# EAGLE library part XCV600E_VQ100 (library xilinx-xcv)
xcv600e_vq100 edit this description Auto generated by make-symbol-device-package-bsdl.ulp Rev. 26 Source: xcv600e_vq100.bsd
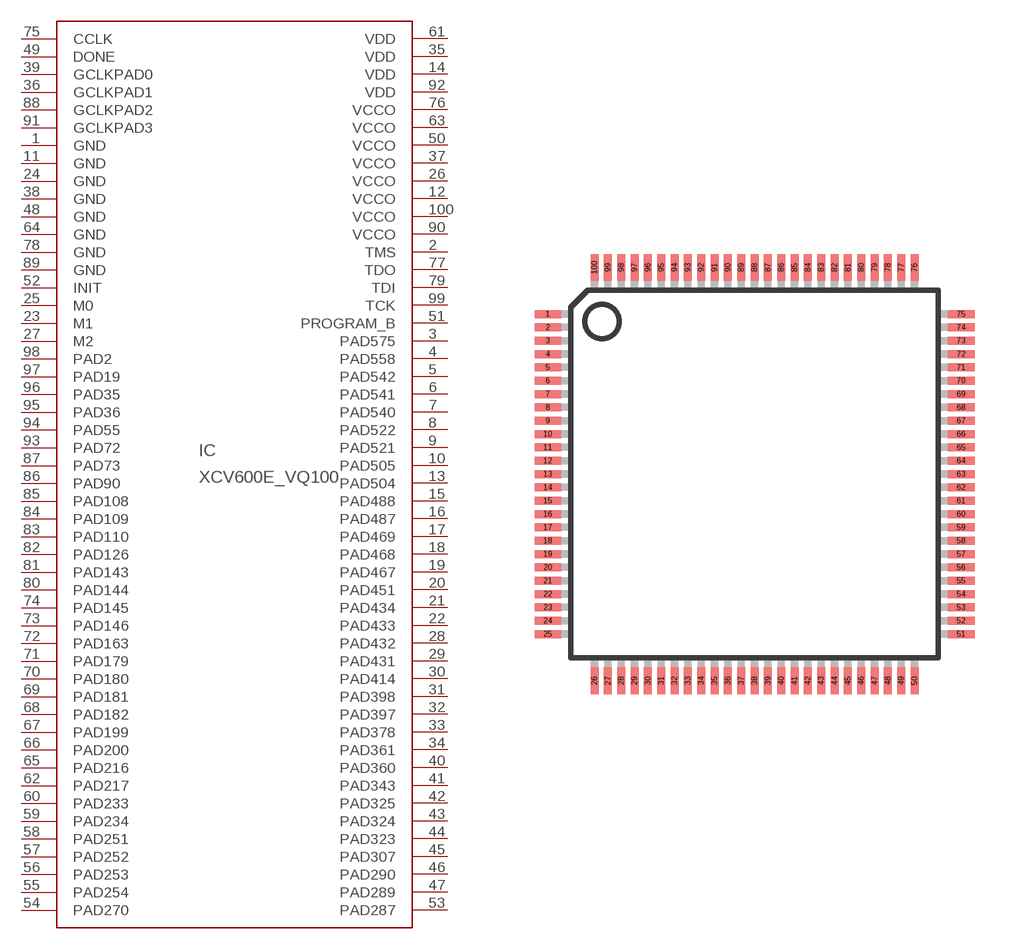
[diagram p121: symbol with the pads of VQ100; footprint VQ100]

Designator prefix IC

## XCV600E_VQ100 (OC_FARNELL: unknown; OC_NEWARK: unknown)  [VQ100]
1  GND  pwr
2  TMS  in
3  PAD575
4  PAD558
5  PAD542
6  PAD541
7  PAD540
8  PAD522
9  PAD521
10  PAD505
11  GND  pwr
12  VCCO  pwr
13  PAD504
14  VDD  pwr
15  PAD488
16  PAD487
17  PAD469
18  PAD468
19  PAD467
20  PAD451
21  PAD434
22  PAD433
23  M1  in
24  GND  pwr
25  M0  in
26  VCCO  pwr
27  M2  in
28  PAD432
29  PAD431
30  PAD414
31  PAD398
32  PAD397
33  PAD378
34  PAD361
35  VDD  pwr
36  GCLKPAD1  in
37  VCCO  pwr
38  GND  pwr
39  GCLKPAD0  in
40  PAD360
41  PAD343
42  PAD325
43  PAD324
44  PAD323
45  PAD307
46  PAD290
47  PAD289
48  GND  pwr
49  DONE
50  VCCO  pwr
51  PROGRAM_B  in
52  INIT
53  PAD287
54  PAD270
55  PAD254
56  PAD253
57  PAD252
58  PAD251
59  PAD234
60  PAD233
61  VDD  pwr
62  PAD217
63  VCCO  pwr
64  GND  pwr
65  PAD216
66  PAD200
67  PAD199
68  PAD182
69  PAD181
70  PAD180
71  PAD179
72  PAD163
73  PAD146
74  PAD145
75  CCLK
76  VCCO  pwr
77  TDO  out
78  GND  pwr
79  TDI  in
80  PAD144
81  PAD143
82  PAD126
83  PAD110
84  PAD109
85  PAD108
86  PAD90
87  PAD73
88  GCLKPAD2  in
89  GND  pwr
90  VCCO  pwr
91  GCLKPAD3  in
92  VDD  pwr
93  PAD72
94  PAD55
95  PAD36
96  PAD35
97  PAD19
98  PAD2
99  TCK  in
100  VCCO  pwr

## Footprint VQ100 (pad centres in mm)
VQ100 Auto generated by make-symbol-device-package-bsdl.ulp Rev. 26
smd 1 x 0.3: 1 -7.75,6; 2 -7.75,5.5; 3 -7.75,5; 4 -7.75,4.5; 5 -7.75,4; 6 -7.75,3.5; 7 -7.75,3; 8 -7.75,2.5; 9 -7.75,2; 10 -7.75,1.5; 11 -7.75,1; 12 -7.75,0.5; 13 -7.75,0; 14 -7.75,-0.5; 15 -7.75,-1; 16 -7.75,-1.5; 17 -7.75,-2; 18 -7.75,-2.5; 19 -7.75,-3; 20 -7.75,-3.5; 21 -7.75,-4; 22 -7.75,-4.5; 23 -7.75,-5; 24 -7.75,-5.5; 25 -7.75,-6; 51 7.75,-6; 52 7.75,-5.5; 53 7.75,-5; 54 7.75,-4.5; 55 7.75,-4; 56 7.75,-3.5; 57 7.75,-3; 58 7.75,-2.5; 59 7.75,-2; 60 7.75,-1.5; 61 7.75,-1; 62 7.75,-0.5; 63 7.75,0; 64 7.75,0.5; 65 7.75,1; 66 7.75,1.5; 67 7.75,2; 68 7.75,2.5; 69 7.75,3; 70 7.75,3.5; 71 7.75,4; 72 7.75,4.5; 73 7.75,5; 74 7.75,5.5; 75 7.75,6
smd 0.3 x 1: 26 -6,-7.75; 27 -5.5,-7.75; 28 -5,-7.75; 29 -4.5,-7.75; 30 -4,-7.75; 31 -3.5,-7.75; 32 -3,-7.75; 33 -2.5,-7.75; 34 -2,-7.75; 35 -1.5,-7.75; 36 -1,-7.75; 37 -0.5,-7.75; 38 0,-7.75; 39 0.5,-7.75; 40 1,-7.75; 41 1.5,-7.75; 42 2,-7.75; 43 2.5,-7.75; 44 3,-7.75; 45 3.5,-7.75; 46 4,-7.75; 47 4.5,-7.75; 48 5,-7.75; 49 5.5,-7.75; 50 6,-7.75; 76 6,7.75; 77 5.5,7.75; 78 5,7.75; 79 4.5,7.75; 80 4,7.75; 81 3.5,7.75; 82 3,7.75; 83 2.5,7.75; 84 2,7.75; 85 1.5,7.75; 86 1,7.75; 87 0.5,7.75; 88 0,7.75; 89 -0.5,7.75; 90 -1,7.75; 91 -1.5,7.75; 92 -2,7.75; 93 -2.5,7.75; 94 -3,7.75; 95 -3.5,7.75; 96 -4,7.75; 97 -4.5,7.75; 98 -5,7.75; 99 -5.5,7.75; 100 -6,7.75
